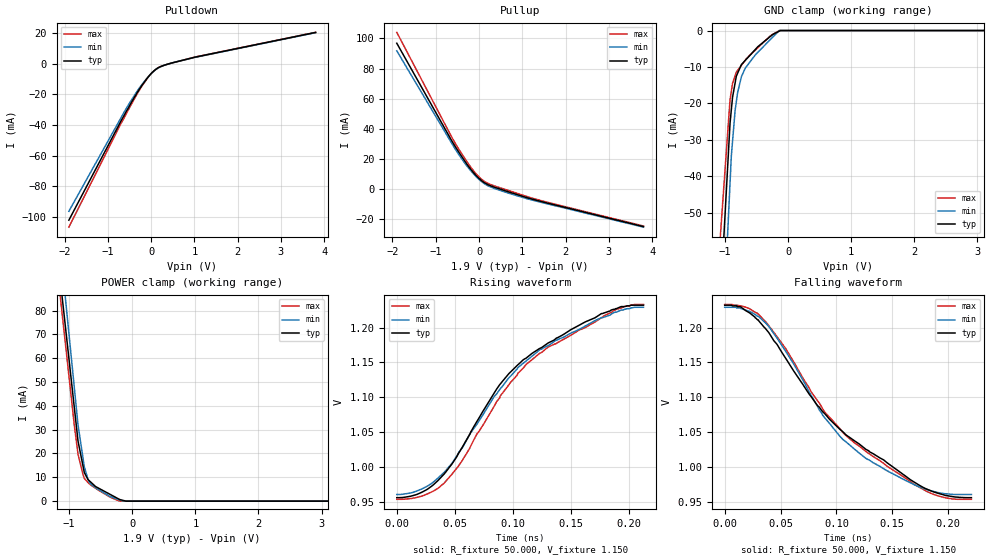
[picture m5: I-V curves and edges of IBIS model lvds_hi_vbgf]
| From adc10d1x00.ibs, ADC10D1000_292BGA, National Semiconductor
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[Model]   lvds_hi_vbgf
Model_type Output
Vref=1.150E+00
Rref=5.000E+01
Cref=0.000E+00
Vmeas=1.150E+00
C_comp   4.84E-13   4.84E-13   4.84E-13
[Voltage Range]   1.900E+00   1.800E+00   2.000E+00
[POWER Clamp Reference]   1.900E+00   1.800E+00   2.000E+00
[GND Clamp Reference]   0.000E+00   0.000E+00   0.000E+00
[Pullup Reference]   1.900E+00   1.800E+00   2.000E+00
[Pulldown Reference]   0.000E+00   0.000E+00   0.000E+00
[Temperature Range]   25   85   -40
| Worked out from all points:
|   slope of the pulldown table from 0 to 0.285 V, typ, clamps not added: 53.7 ohm
|   slope of the pullup table from 0 to 0.285 V, typ, clamps not added: 56 ohm
|   GND clamp passes 1 mA (typ) near -0.24 V on its own axis
|   POWER clamp passes 1 mA (typ) near -0.22 V on its own axis
|   rising waveform, R_fixture 50.000, V_fixture 1.150: 20-80 % time 79.3ps typ, 80.7ps min, 81.3ps max; typ from 0.956 V to 1.23 V
|   falling waveform, R_fixture 50.000, V_fixture 1.150: 20-80 % time 94.7ps typ, 74.1ps min, 87.2ps max; typ from 1.23 V to 0.956 V
[GND Clamp]
-2V       -368.8mA   -437.3mA   -281.6mA
-1.8V     -305.2mA   -364mA     -232.9mA
-920mV    -25.41mA   -41.86mA   -19.01mA
-900mV    -21.84mA   -34.54mA   -16.75mA
-880mV    -18.27mA   -30.36mA   -14.49mA
-840mV    -14.43mA   -21.99mA   -12.43mA
-800mV    -11.72mA   -17.02mA   -10.94mA
-740mV    -9.361mA   -12.67mA   -9.542mA
-680mV    -8.227mA   -10.36mA   -8.148mA
-520mV    -5.203mA   -6.699mA   -5.383mA
-140mV    -173.1uA   0A         0A
4V        0A         0A         0A
[POWER Clamp]
-2.1V     323.5mA    363.2mA    318.9mA
-1.7V     227.3mA    255.8mA    221.7mA
-980mV    54.15mA    64.06mA    46.82mA
-920mV    39.72mA    48.08mA    32.25mA
-860mV    25.29mA    32.1mA     19.78mA
-760mV    12.02mA    14.43mA    9.543mA
-700mV    9.016mA    8.989mA    7.766mA
-660mV    8.043mA    7.222mA    6.814mA
-360mV    2.964mA    2.076mA    1.818mA
-200mV    684.4uA    475.1uA    0A
-100mV    0A         0A         0A
3.9V      0A         0A         0A
[Pullup]
-1.9V     96.8mA     91.77mA    104mA
-540mV    27.86mA    26.16mA    29.98mA
-340mV    19.09mA    17.71mA    20.93mA
-180mV    12.8mA     11.9mA     14.21mA
-60mV     8.879mA    8.13mA     9.93mA
100mV     4.778mA    4.124mA    5.661mA
200mV     3.101mA    2.368mA    3.946mA
400mV     916uA      60.01uA    1.759mA
1.08V     -5.366mA   -6.072mA   -4.6mA
1.74V     -10.33mA   -10.83mA   -9.824mA
3.8V      -24.81mA   -25.16mA   -24.42mA
[Pulldown]
-1.9V     -102.1mA   -96.29mA   -106.6mA
-700mV    -37.62mA   -35.47mA   -39.3mA
-460mV    -25.49mA   -23.94mA   -26.65mA
-240mV    -15.29mA   -14.58mA   -15.8mA
-100mV    -9.804mA   -9.572mA   -9.977mA
0V        -6.456mA   -6.47mA    -6.458mA
100mV     -3.853mA   -3.979mA   -3.792mA
320mV     -807.4uA   -839.7uA   -818.3uA
1V        4.194mA    4.063mA    4.265mA
3.8V      20.43mA    20.28mA    20.51mA
[Rising Waveform]
R_fixture = 50.000
V_fixture = 1.150
V_fixture_min = 1.150
V_fixture_max = 1.150
|  time   V(typ)   V(min)   V(max)
0s        955.8mV    960.4mV    953.5mV
22.25ps   964.2mV    969mV      958.4mV
40.5ps    989.2mV    991.6mV    976.2mV
56.75ps   1.029V     1.028V     1.01V
88.75ps   1.118V     1.111V     1.099V
109.2ps   1.154V     1.149V     1.142V
130.7ps   1.178V     1.174V     1.172V
176.5ps   1.22V      1.214V     1.214V
196.2ps   1.23V      1.226V     1.23V
212.7ps   1.232V     1.229V     1.233V
[Falling Waveform]
R_fixture = 50.000
V_fixture = 1.150
V_fixture_min = 1.150
V_fixture_max = 1.150
|  time   V(typ)   V(min)   V(max)
0s        1.232V     1.229V     1.233V
14.75ps   1.229V     1.227V     1.231V
28.75ps   1.212V     1.217V     1.221V
39.75ps   1.192V     1.201V     1.202V
62ps      1.137V     1.147V     1.15V
87.75ps   1.079V     1.074V     1.083V
106ps     1.05V      1.039V     1.049V
126.5ps   1.025V     1.012V     1.022V
181.5ps   967.7mV    967.3mV    964.2mV
220.7ps   955.8mV    960.4mV    953.5mV
[Ramp]
dV/dt_r   1.7621E+00/7.9160E-11   1.7024E+00/8.0480E-11   1.8222E+00/8.0750E-11
dV/dt_f   1.7621E+00/9.4438E-11   1.7024E+00/7.4086E-11   1.8222E+00/8.6703E-11
R_load = 50
